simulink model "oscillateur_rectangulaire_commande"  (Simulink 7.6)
settings: Solver=ode15s  StartTime=0.0  StopTime=2  RelTol=1e-3
undefined symbols (not defined in the file or in its folder): sigbuilder_block
libraries: fl_lib x6, elec_lib x5, nesl_utility x3

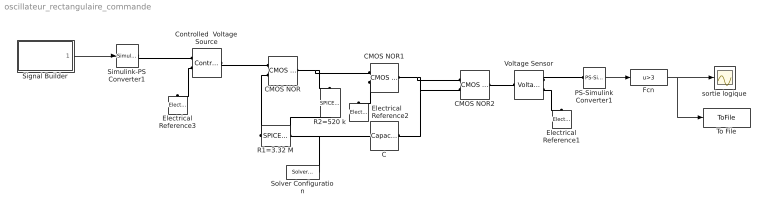
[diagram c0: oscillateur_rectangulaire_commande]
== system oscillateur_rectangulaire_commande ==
  C : fl_lib/Electrical/Electrical Elements/Capacitor  DialogController=NetworkEngine.DynNeDlgSource  SystemSampleTime=-1  c=0.1 uF  v0=0 V  r=1e-6 Ohm  g=0 1/Ohm  i_Log=off  v_Log=off  vc_Log=off  LocalVarNames=|current|voltage|power  LocalVarDescs=|Capacitor current (A)|Voltage across capacitor (V)|Power (W)  LocalVarLogging=[0 0 0]
  CMOS NOR : elec_lib/Integrated Circuits/Logic/CMOS NOR  DialogController=NetworkEngine.DynNeDlgSource  SystemSampleTime=-1  V_IL=2 V  V_IH=3 V  C_IN=5 pF  output_type=1  V_OL=0 V  V_OH=5 V  V_CC=5 V  V_meas=5 V  R_OUT=450 Ohm  R_OH=[ 25 250 ] Ohm  I_OH=63 mA  R_OL=[ 30 800 ] Ohm  I_OL=-45 mA  Delay=1.2e-07 s  Ron=5 Ohm  Vf=0.6 V  output_state=1  LocalVarLogging=[]
  CMOS NOR1 : elec_lib/Integrated Circuits/Logic/CMOS NOR  DialogController=NetworkEngine.DynNeDlgSource  SystemSampleTime=-1  V_IL=2 V  V_IH=3 V  C_IN=5 pF  output_type=1  V_OL=0 V  V_OH=5 V  V_CC=5 V  V_meas=5 V  R_OUT=450 Ohm  R_OH=[ 25 250 ] Ohm  I_OH=63 mA  R_OL=[ 30 800 ] Ohm  I_OL=-45 mA  Delay=1.2e-07 s  Ron=5 Ohm  Vf=0.6 V  output_state=1  LocalVarLogging=[]
  CMOS NOR2 : elec_lib/Integrated Circuits/Logic/CMOS NOR  DialogController=NetworkEngine.DynNeDlgSource  SystemSampleTime=-1  V_IL=2 V  V_IH=3 V  C_IN=5 pF  output_type=1  V_OL=0 V  V_OH=5 V  V_CC=5 V  V_meas=5 V  R_OUT=450 Ohm  R_OH=[ 25 250 ] Ohm  I_OH=63 mA  R_OL=[ 30 800 ] Ohm  I_OL=-45 mA  Delay=1.2e-07 s  Ron=5 Ohm  Vf=0.6 V  output_state=1  LocalVarLogging=[]
  Controlled  Voltage Source : fl_lib/Electrical/Electrical Sources/Controlled Voltage Source  DialogController=NetworkEngine.DynNeDlgSource  SystemSampleTime=-1  i_Log=off  v_Log=off  LocalVarNames=|i|v  LocalVarDescs=|i|v  LocalVarLogging=[0 0]
  Electrical Reference1 : fl_lib/Electrical/Electrical Elements/Electrical Reference  DialogController=NetworkEngine.DynNeDlgSource  SystemSampleTime=-1  i_Log=off  LocalVarNames=|i  LocalVarDescs=|i  LocalVarLogging=[]
  Electrical Reference2 : fl_lib/Electrical/Electrical Elements/Electrical Reference  DialogController=NetworkEngine.DynNeDlgSource  SystemSampleTime=-1  i_Log=off  LocalVarNames=|i  LocalVarDescs=|i  LocalVarLogging=[]
  Electrical Reference3 : fl_lib/Electrical/Electrical Elements/Electrical Reference  DialogController=NetworkEngine.DynNeDlgSource  SystemSampleTime=-1  i_Log=off  LocalVarNames=|i  LocalVarDescs=|i  LocalVarLogging=[]
  Fcn : Fcn  Expr=u>3
  PS-Simulink Converter1 : nesl_utility/PS-Simulink Converter  DialogController=NetworkEngine.DynNeUtilDlgSource  SystemSampleTime=-1  PhysicalDomain=network_engine_domain  LeftPortType=input  RightPortType=output  SubClassName=ps_output  Unit=1  AffineConversion=off
  R1=3.32 M : elec_lib/Additional Components/SPICE-Compatible Components/Passive Devices/SPICE Resistor  DialogController=NetworkEngine.DynNeDlgSource  SystemSampleTime=-1  SCALE=1  R_param=1  R=2.2 MOhm  RSH=0 Ohm  LENGTH=1e-06 m  WIDTH=1e-06 m  NARROW=0 m  T_param=1  TC1=0 1/K  TC2=0 1/K^2  TOFFSET=0 K  TFIXED=300.15 K  TMEAS=300.15 K  LocalVarLogging=[]
  R2=520 k : elec_lib/Additional Components/SPICE-Compatible Components/Passive Devices/SPICE Resistor  DialogController=NetworkEngine.DynNeDlgSource  SystemSampleTime=-1  SCALE=1  R_param=1  R=470 kOhm  RSH=0 Ohm  LENGTH=1e-06 m  WIDTH=1e-06 m  NARROW=0 m  T_param=1  TC1=0 1/K  TC2=0 1/K^2  TOFFSET=0 K  TFIXED=300.15 K  TMEAS=300.15 K  LocalVarLogging=[]
  Signal Builder : Subsystem  Tag=STV Subsys  LoadFcn=sigbuilder_block('load',[198 37.5 550.5 399.75 ]);  StartFcn=sigbuilder_block('start');  StopFcn=sigbuilder_block('stop');  ClipboardFcn=sigbuilder_block('clipboard');
  Simulink-PS Converter1 : nesl_utility/Simulink-PS Converter  DialogController=NetworkEngine.DynNeUtilDlgSource  SystemSampleTime=-1  PhysicalDomain=network_engine_domain  LeftPortType=input  RightPortType=output  SubClassName=ps_input  Unit=1  AffineConversion=off  InputFilterTimeConstant=.001  UdotUserProvided=0
  Solver Configuration : nesl_utility/Solver Configuration  DialogController=NetworkEngine.DynNeUtilDlgSource  SystemSampleTime=-1  PhysicalDomain=network_engine_domain  LeftPortType=input  RightPortType=generic  SubClassName=solver  Accelerate=off  Profile=off  ResidualTolerance=1e-9  MaxNonlinIter=12  MaxModeIter=2  DoFixedCost=off  UseLocalSampling=off  DoDC=off  LinearAlgebra=Sparse  LocalSolverSampleTime=.001  LocalSolverChoice=NE_BACKWARD_EULER_ADVANCER  UseLocalSolver=off
  To File : ToFile  Filename=signaux  MatrixName=x
  Voltage Sensor : fl_lib/Electrical/Electrical Sensors/Voltage Sensor  DialogController=NetworkEngine.DynNeDlgSource  SystemSampleTime=-1  i1_Log=off  v1_Log=off  LocalVarNames=|i1|v1  LocalVarDescs=|i1|v1  LocalVarLogging=[0 0]
  sortie logique : Scope
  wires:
  PS-Simulink Converter1/1 -> Fcn/1
  Fcn/1 -> To File/1, sortie logique/1
  Signal Builder/1(Signal 1) -> Simulink-PS Converter1/1
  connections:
  Voltage Sensor/RConn1 -- PS-Simulink Converter1/LConn1
  Voltage Sensor/RConn2 -- Electrical Reference1/LConn1
  CMOS NOR1/LConn2 -- Electrical Reference2/LConn1
  CMOS NOR/RConn1 -- R2=520 k/LConn1 -- CMOS NOR1/LConn1
  CMOS NOR/LConn2 -- R1=3.32 M/LConn1
  R1=3.32 M/RConn1 -- R2=520 k/RConn1 -- C/RConn1 -- Solver Configuration/RConn1
  C/LConn1 -- CMOS NOR1/RConn1 -- CMOS NOR2/LConn1 -- CMOS NOR2/LConn2
  Controlled  Voltage Source/LConn1 -- CMOS NOR/LConn1
  Simulink-PS Converter1/RConn1 -- Controlled  Voltage Source/RConn1
  Controlled  Voltage Source/RConn2 -- Electrical Reference3/LConn1
  Voltage Sensor/LConn1 -- CMOS NOR2/RConn1

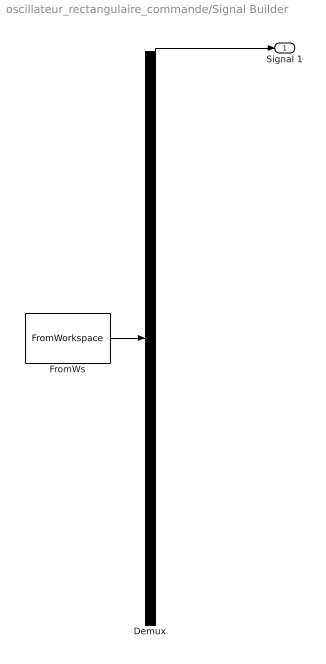
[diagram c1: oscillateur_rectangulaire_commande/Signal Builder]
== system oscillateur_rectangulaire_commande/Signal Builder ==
  Demux : Demux  Tag=STV Demux  Outputs=1
  FromWs : FromWorkspace  Tag=STV FromWs  VariableName=tuvar  SampleTime=0  SigBuilderData=DataTag0  VnvData=DataTag1
  Signal 1 : Outport  Tag=STV Outport
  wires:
  FromWs/1 -> Demux/1
  Demux/1 -> Signal 1/1
